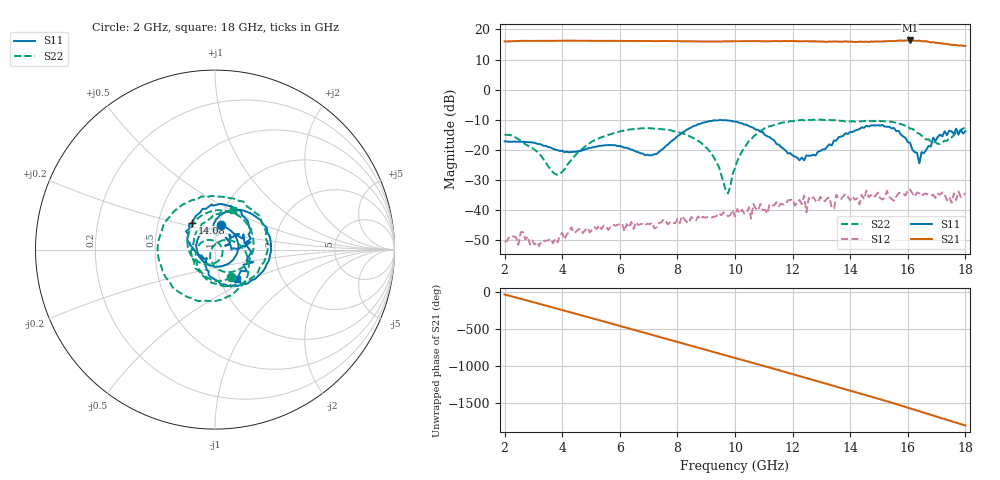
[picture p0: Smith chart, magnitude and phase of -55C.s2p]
!Agilent Technologies,N5230A,MY45001466,A.07.50.67
!Agilent N5230A: A.07.50.67
!Date: Monday, February 09, 2026 16:40:54
!Correction: S11(Full 2 Port(1,2))
!S21(Full 2 Port(1,2))
!S12(Full 2 Port(1,2))
!S22(Full 2 Port(1,2))
!S2P File: Measurements: S11, S21, S12, S22:
# Hz S  dB  R 50
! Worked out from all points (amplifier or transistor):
!   201 points, 2 GHz to 18 GHz, reference 50 ohm
!   highest |S21| = 16.4 dB at 16.08 GHz (marker M1)
!   |S21| within 3 dB of that: start of sweep to end of sweep
!   unconditionally stable (mu >= 1): start of sweep to end of sweep
!   at 4.64 GHz: K = 15.43, MAG = 16.4 dB, |S12| = -46.2 dB
!   at 10 GHz: K = 9.06, MAG = 16.5 dB, |S12| = -42.1 dB
!   at 18 GHz: K = 4.42, MAG = 15.0 dB, |S12| = -34.4 dB
!   S11 on the Smith chart (normalised r, x): 2 GHz: 1.02, +0.28; 14.08 GHz: 0.74, +0.23; 18 GHz: 1.19, -0.41
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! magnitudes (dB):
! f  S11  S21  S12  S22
! 2 GHz  -17.1  16.1  -50.6  -15.0
! 2.48 GHz  -17.2  16.2  -51.5  -16.4
! 2.56 GHz  -17.3  16.2  -47.3  -16.9
! 3.84 GHz  -20.1  16.2  -50.7  -28.2
! 4.32 GHz  -20.6  16.3  -45.6  -23.2
! 4.72 GHz  -20.0  16.2  -47.6  -19.4
! 7.36 GHz  -20.6  16.2  -44.2  -13.0
! 8.88 GHz  -11.0  16.0  -42.2  -18.1
! 9.76 GHz  -10.2  16.1  -42.0  -34.4
! 10 GHz  -10.6  16.1  -42.1  -25.9
! 11.04 GHz  -15.0  16.1  -39.8  -12.7
! 12.4 GHz  -23.4  16.1  -35.1  -10.2
! 12.48 GHz  -21.8  16.1  -40.7  -10.0
! 12.72 GHz  -21.6  16.1  -35.7  -9.9
! 13.44 GHz  -16.8  16.0  -39.4  -10.1
! 13.52 GHz  -16.9  16.0  -34.8  -10.2
! 14.08 GHz  -14.0  15.9  -35.4  -10.5
! 15.36 GHz  -12.3  16.2  -35.6  -10.6
! 16.08 GHz  -17.6  16.4  -33.1  -12.9
! 16.4 GHz  -24.4  16.3  -34.4  -14.6
! 16.88 GHz  -15.9  15.8  -34.9  -17.5
! 18 GHz  -13.8  14.5  -34.4  -12.3
